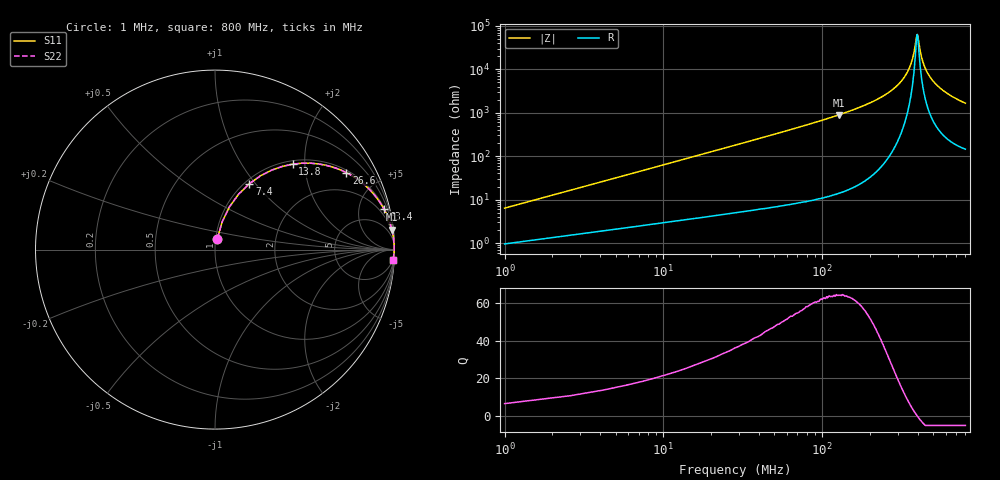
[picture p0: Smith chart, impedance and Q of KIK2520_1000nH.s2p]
!version-2
!date-01.2022
!Series
# MHz S RI R 50
!Freq ReS11 ImS11 ReS21 ImS21 ReS12 ImS12 ReS22 ImS22
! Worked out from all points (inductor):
!   501 points, 1 MHz to 800 MHz, reference 50 ohm
!   read as one part in series: L = 1 uH near 4.2 MHz
!   highest Q = 64.1 at 127 MHz (marker M1), where L = 1.12 uH
!   self-resonance near 398 MHz
!   S11 on the Smith chart (normalised r, x): 1 MHz: 1.02, +0.13; 7.4 MHz: 1.05, +0.93; 13.8 MHz: 1.07, +1.74; 26.6 MHz: 1.10, +3.36; 63.4 MHz: 1.15, +8.17; 800 MHz: 4, -33
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1  0.0132 0.0614  0.9867 -0.0614  0.9867 -0.0614  0.0132 0.0614
5.8  0.1322 0.3094  0.8678 -0.3094  0.8678 -0.3094  0.1322 0.3094
7.4  0.1911 0.3669  0.8089 -0.3669  0.8089 -0.3669  0.1911 0.3669
13.8  0.4328 0.476  0.5672 -0.476  0.5672 -0.476  0.4328 0.476
26.6  0.7324 0.4286  0.2676 -0.4286  0.2676 -0.4286  0.7324 0.4286
41  0.8658 0.3294  0.1342 -0.3294  0.1342 -0.3294  0.8658 0.3294
63.4  0.9397 0.2288  0.0603 -0.2288  0.0603 -0.2288  0.9397 0.2288
127  0.9859 0.1103  0.0141 -0.1103  0.0141 -0.1103  0.9859 0.1103
135  0.9877 0.1025  0.0123 -0.1025  0.0123 -0.1025  0.9877 0.1025
268  0.9978 0.0323  0.00216 -0.0323  0.00216 -0.0323  0.9978 0.0323
315  0.9984 0.0189  0.00158 -0.0189  0.00158 -0.0189  0.9984 0.0189
347  0.9985 0.0111  0.00146 -0.0111  0.00146 -0.0111  0.9985 0.0111
371  0.9985 0.0057  0.00147 -0.0057  0.00147 -0.0057  0.9985 0.0057
379  0.9985 0.004  0.00149 -0.004  0.00149 -0.004  0.9985 0.004
396  0.9984 0.000378  0.00157 -0.000378  0.00157 -0.000378  0.9984 0.000378
401  0.9984 -0.000581  0.00159 0.000581  0.00159 0.000581  0.9984 -0.000581
423  0.9983 -0.00491  0.00174 0.00491  0.00174 0.00491  0.9983 -0.00491
447  0.998 -0.00931  0.00195 0.00931  0.00195 0.00931  0.998 -0.00931
487  0.9976 -0.0162  0.0024 0.0162  0.0024 0.0162  0.9976 -0.0162
534  0.9969 -0.0236  0.00305 0.0236  0.00305 0.0236  0.9969 -0.0236
667  0.9945 -0.0425  0.00555 0.0425  0.00555 0.0425  0.9945 -0.0425
800  0.9912 -0.0593  0.00881 0.0593  0.00881 0.0593  0.9912 -0.0593
